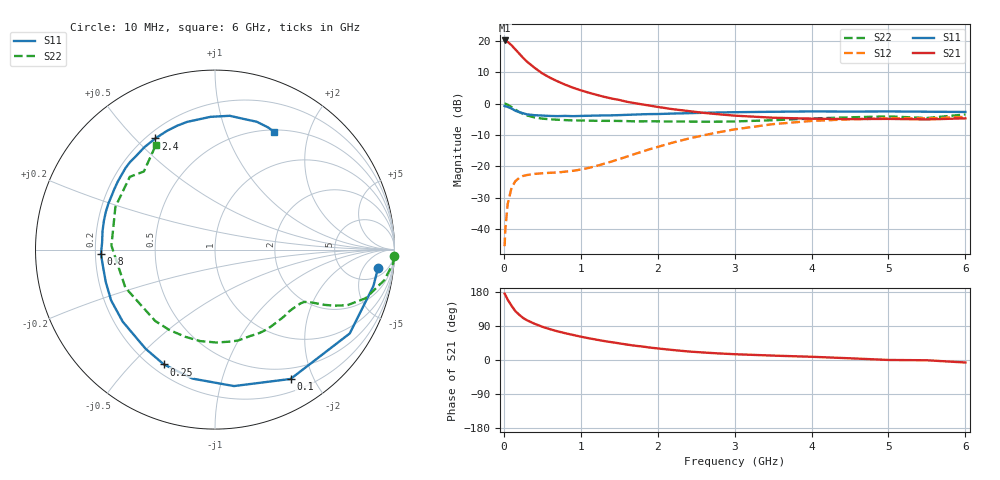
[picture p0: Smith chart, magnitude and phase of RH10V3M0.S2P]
! SIEMENS Small Signal Semiconductors
! BFR106
! Si NPN RF Bipolar Junction Transistor in SOT23
! VCE = 10 V  IC = 3 mA
! Common Emitter S-Parameters:  August  1996
# GHz  S  MA  R  50
!  f  S11  S21  S12  S22
! GHz  MAG  ANG  MAG  ANG  MAG  ANG  MAG  ANG
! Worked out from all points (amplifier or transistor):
!   36 points, 10 MHz to 6 GHz, reference 50 ohm
!   highest |S21| = 20.2 dB at 10 MHz (marker M1)
!   |S21| within 3 dB of that: start of sweep to 154.8 MHz
!   unconditionally stable (mu >= 1): 714.4 MHz to 1.817 GHz; 4.463 GHz to end of sweep
!   at 250 MHz: K = 0.38, MSG = 18.9 dB, |S12| = -23.1 dB
!   at 1.4 GHz: K = 1.19, MAG = 7.4 dB, |S12| = -18.5 dB
!   at 6 GHz: K = 1.02, MAG = -1.1 dB, |S12| = -4.2 dB
!   S11 on the Smith chart (normalised r, x): 10 MHz: 9, -11; 100 MHz: 0.35, -1.69; 250 MHz: 0.25, -0.62; 800 MHz: 0.22, -0.02; 2.4 GHz: 0.23, +0.57; 6 GHz: 0.52, +1.49
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0.01  0.914 -6.4  10.18 175.1  0.0053 88.1  0.9982 -2.2
0.02  0.9058 -12.9  10.1 171.8  0.0102 81.6  0.9952 -4.4
0.05  0.8842 -31.9  9.645 159.3  0.025 73.1  0.9588 -10.2
0.1  0.8347 -59.7  8.536 143.2  0.0452 60.1  0.8822 -17.9
0.15  0.7676 -82.1  7.309 128.8  0.0579 49.2  0.7996 -22.8
0.2  0.7296 -99.8  6.285 119.4  0.0651 43.5  0.734 -25.2
0.25  0.7003 -114.0  5.379 111.0  0.07 38.8  0.6823 -26.8
0.3  0.6743 -125.0  4.683 105.0  0.0723 36.7  0.648 -27.7
0.4  0.6523 -142.0  3.722 95.6  0.0755 33.8  0.6002 -29.1
0.5  0.6443 -153.9  3.035 87.7  0.0772 34.0  0.575 -30.5
0.6  0.6349 -163.4  2.589 81.3  0.0786 35.7  0.5616 -32.4
0.8  0.6359 -177.7  1.997 70.6  0.082 41.7  0.5447 -37.1
1.1  0.6396 165.3  1.498 57.6  0.0938 54.4  0.5336 -45.9
1.6  0.6611 145.0  1.069 40.7  0.1426 68.4  0.5254 -63.5
2.2  0.6931 124.5  0.813 26.3  0.2391 68.7  0.5178 -89.0
2.4  0.7028 118.2  0.76 22.5  0.2761 66.4  0.5163 -99.2
3  0.7284 102.3  0.642 15.3  0.3876 55.4  0.5188 -130.0
3.5  0.7402 91.9  0.595 11.6  0.4703 44.2  0.5426 -157.0
4.5  0.7453 77.3  0.566 4.5  0.5612 22.0  0.6038 156.8
5  0.7493 72.0  0.57 0.1  0.5795 13.0  0.6243 139.5
5.5  0.7421 66.5  0.558 -0.7  0.5803 8.4  0.5886 132.3
6  0.7345 63.3  0.582 -6.6  0.6136 0.2  0.6701 119.4
